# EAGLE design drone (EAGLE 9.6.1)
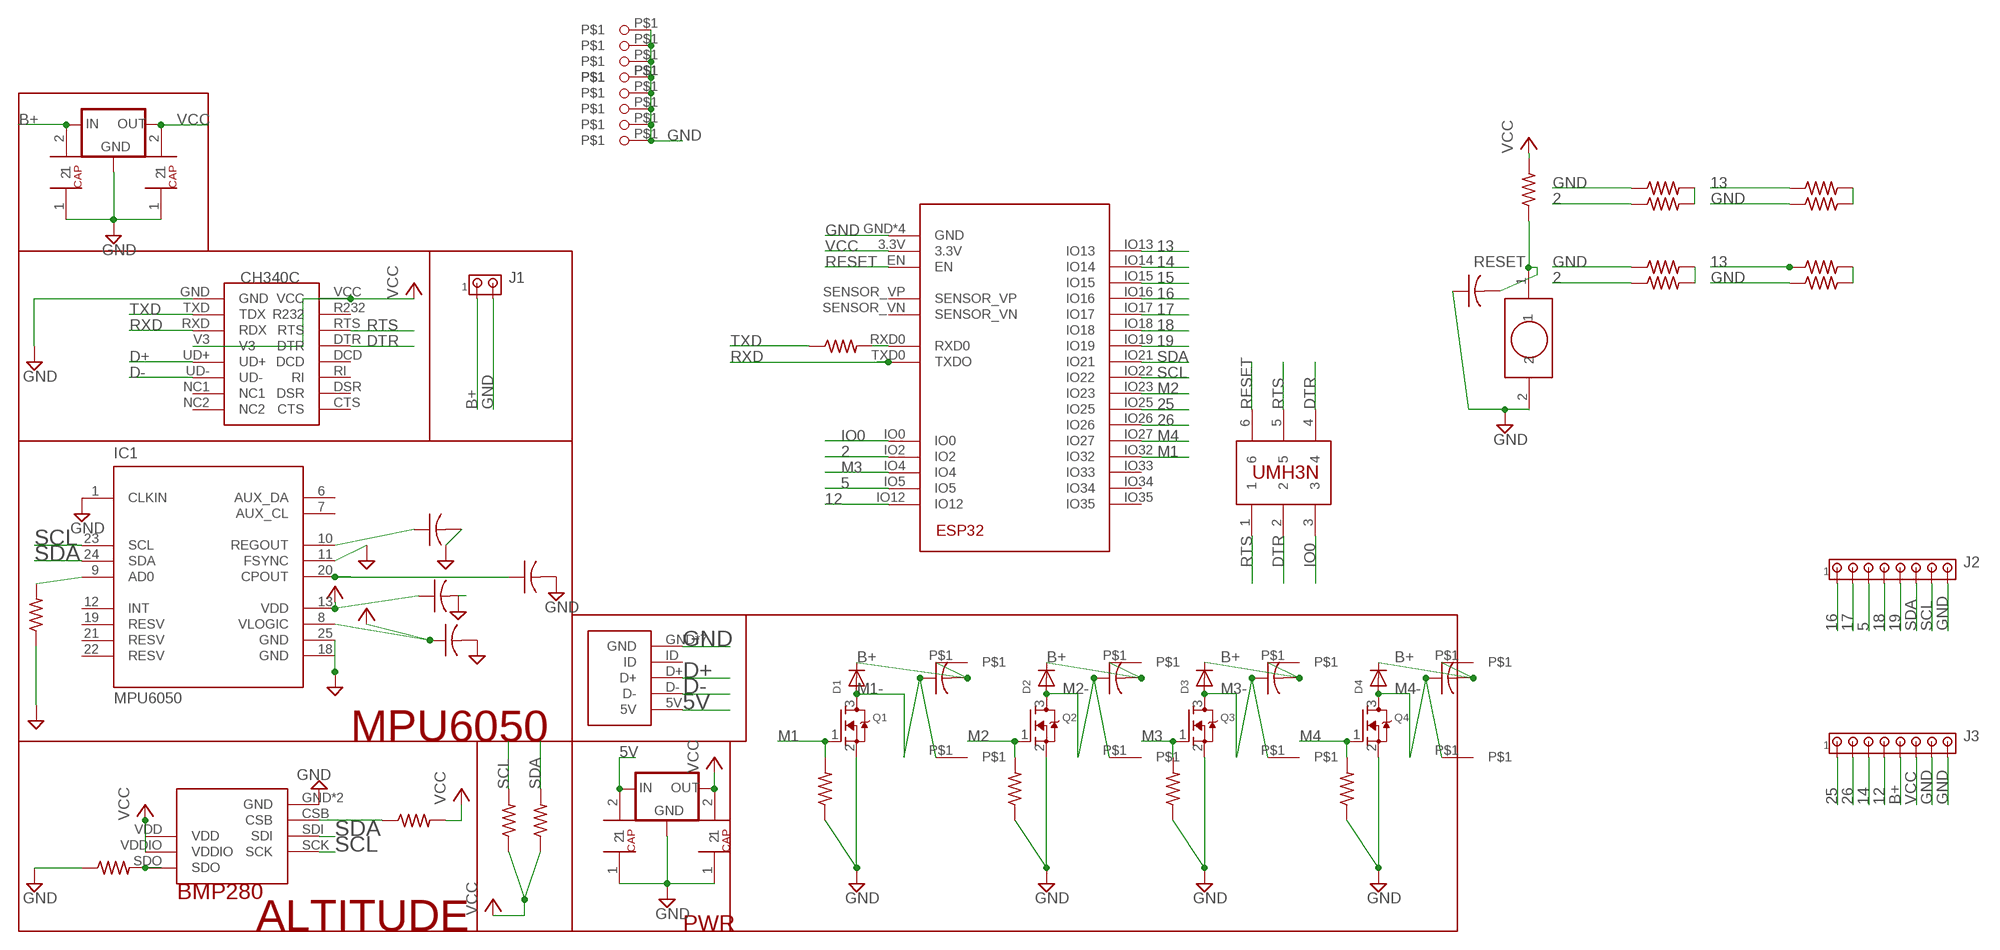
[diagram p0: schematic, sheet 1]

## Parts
D1  DIODESOD-323F  [SOD-323F]
D2  DIODESOD-323F  [SOD-323F]
D3  DIODESOD-323F  [SOD-323F]
D4  DIODESOD-323F  [SOD-323F]
IC1  MPU6050  [QFN50P400X400X95-25T265X275N]
IC2  SELF_VREG3.3MP  [SOT223]
IC3  SELF_VREG3.3MP  [SOT223]
J1  MTA02-100  [10X02MTA]
J2  MTA08-100  [10X08MTA]
J3  MTA08-100  [10X08MTA]
Q1  MOSFET-NREFLOW  [SOT23]
Q2  MOSFET-NREFLOW  [SOT23]
Q3  MOSFET-NREFLOW  [SOT23]
Q4  MOSFET-NREFLOW  [SOT23]
U1  ESP32  [MODULE_ESP-WROOM-32]
U$1  MICROUSB  [USB]
U$2  CH340C  [SOIC16]
U$3  BMP280  [BMP280]
U$4  R-US_R0603  [R0603]
U$5  R-US_R0603  [R0603]
U$6  C-USC0603  [C0603]
U$7  R-US_R0603  [R0603]
U$8  C-USC0603  [C0603]
U$9  C-USC0603  [C0603]
U$10  C-USC0603  [C0603]
U$11  R-US_R0603  [R0603]
U$12  R-US_R0603  [R0603]
U$13  SELF_CAP_0603SELF_CAP_0805  [SELF_CAP_0805]
U$14  SELF_CAP_0603SELF_CAP_0805  [SELF_CAP_0805]
U$16  R-US_R0603  [R0603]
U$18  SELF_CAP_0603SELF_CAP_0805  [SELF_CAP_0805]
U$19  SELF_CAP_0603SELF_CAP_0805  [SELF_CAP_0805]
U$20  R-US_R0603  [R0603]
U$21  R-US_R0603  [R0603]
U$22  R-US_R0603  [R0603]
U$23  R-US_R0603  [R0603]
U$24  C-USC0603  [C0603]
U$25  C-USC0603  [C0603]
U$26  C-USC0603  [C0603]
U$27  C-USC0603  [C0603]
U$28  UMH3N  [UMH3N]
U$29  SELF_PUSHBUTTON  [SELF_PUSHBUTTON]
U$30  R-US_R0603  [R0603]
U$31  C-USC0603  [C0603]
U$32  R-US_R0603  [R0603]
U$33  R-US_R0603  [R0603]
U$34  R-US_R0603  [R0603]
U$35  R-US_R0603  [R0603]
U$36  R-US_R0603  [R0603]
U$37  R-US_R0603  [R0603]
U$38  R-US_R0603  [R0603]
U$39  R-US_R0603  [R0603]
U$40  SELF_PINOUTS  [PINOUTS]
U$41  SELF_PINOUTS  [PINOUTS]
U$42  SELF_PINOUTS  [PINOUTS]
U$43  SELF_PINOUTS  [PINOUTS]
U$44  SELF_PINOUTS  [PINOUTS]
U$45  SELF_PINOUTS  [PINOUTS]
U$46  SELF_PINOUTS  [PINOUTS]
U$47  SELF_PINOUTS  [PINOUTS]
U$48  SELF_PIN2  [PIN2]
U$49  SELF_PIN2  [PIN2]
U$50  SELF_PIN2  [PIN2]
U$51  SELF_PIN2  [PIN2]
U$52  SELF_PIN2  [PIN2]
U$53  SELF_PIN2  [PIN2]
U$54  SELF_PIN2  [PIN2]
U$55  SELF_PIN2  [PIN2]
U$56  SELF_PIN2  [PIN2]

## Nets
2: U1.IO2 U$33.1 U$39.1
5: J2.3 U1.IO5
5V: IC2.VIN(IN) U$1.5V U$13.2
12: J3.4 U1.IO12
13: U1.IO13 U$34.1 U$36.1
14: J3.3 U1.IO14
15: U1.IO15
16: J2.1 U1.IO16
17: J2.2 U1.IO17
18: J2.4 U1.IO18
19: J2.5 U1.IO19
25: J3.1 U1.IO25
26: J3.2 U1.IO26
B+: D1.C D2.C D3.C D4.C IC3.VIN(IN) J1.1 J3.5 U$19.2 U$24.2 U$25.2 U$26.2 U$27.2 U$40.P$1 U$42.P$1 U$44.P$1 U$46.P$1
D+: U$1.D+ U$2.UD+
D-: U$1.D- U$2.UD-
DTR: U$2.DTR U$28.2 U$28.4
GND: IC1.1(CLKIN) IC1.11(FSYNC) IC1.18(GND) IC1.25(GND) IC2.GND IC3.GND J1.2 J2.8 J3.7 J3.8 Q1.2(S) Q2.2(S) Q3.2(S) Q4.2(S) U1.GND U1.GND1(GND) U1.GND2(GND) U1.GND3(GND) U$1.GND U$1.GND1(GND) U$1.GND2(GND) U$1.GND3(GND) U$1.GND4(GND) U$1.GND5(GND) U$1.GND6(GND) U$2.GND U$3.GND U$3.GND1(GND) U$5.1 U$6.2 U$7.1 U$8.2 U$9.2 U$10.2 U$13.1 U$14.1 U$18.1 U$19.1 U$20.1 U$21.1 U$22.1 U$23.1 U$29.2 U$31.1 U$32.1 U$35.1 U$37.1 U$38.1 U$48.P$1 U$49.P$1 U$50.P$1 U$51.P$1 U$52.P$1 U$53.P$1 U$54.P$1 U$55.P$1 U$56.P$1
IO0: U1.IO0 U$28.3
M1: Q1.1(G) U1.IO32 U$20.2
M1-: D1.A Q1.3(D) U$24.1 U$41.P$1
M2: Q2.1(G) U1.IO23 U$21.2
M2-: D2.A Q2.3(D) U$26.1 U$43.P$1
M3: Q3.1(G) U1.IO4 U$22.2
M3-: D3.A Q3.3(D) U$27.1 U$45.P$1
M4: Q4.1(G) U1.IO27 U$23.2
M4-: D4.A Q4.3(D) U$25.1 U$47.P$1
N$1: U$32.2 U$33.2
N$2: U$38.2 U$39.2
N$4: U$34.2 U$35.2
N$5: U$36.2 U$37.2
N$13: U$3.SDO U$5.2
N$14: U$3.CSB U$4.1
N$15: IC1.9(AD0) U$7.2
N$16: IC1.10(REGOUT) U$8.1
N$17: IC1.20(CPOUT) U$10.1
N$18: U1.RXD0 U$16.2
RESET: U1.EN U$28.6 U$29.1 U$30.1 U$31.2
RTS: U$2.RTS U$28.1 U$28.5
RXD: U1.TXD0(TXDO) U$2.RXD(RDX)
SCL: IC1.23(SCL) J2.7 U1.IO22 U$3.SCK U$11.2
SDA: IC1.24(SDA) J2.6 U1.IO21 U$3.SDI U$12.2
TXD: U$2.TXD(TDX) U$16.1
VCC: IC1.8(VLOGIC) IC1.13(VDD) IC2.VOUT1(OUT) IC2.VOUT(OUT) IC3.VOUT1(OUT) IC3.VOUT(OUT) J3.6 U1.3.3V U$2.V3 U$2.VCC U$3.VDD U$3.VDDIO U$4.2 U$6.1 U$9.1 U$11.1 U$12.1 U$14.2 U$18.2 U$30.2
Unconnected: IC1.2(NC) IC1.3(NC) IC1.4(NC) IC1.5(NC) IC1.6(AUX_DA) IC1.7(AUX_CL) IC1.12(INT) IC1.14(NC) IC1.15(NC) IC1.16(NC) IC1.17(NC) IC1.19(RESV) IC1.21(RESV) IC1.22(RESV) U1.IO33 U1.IO34 U1.IO35 U1.SENSOR_VN U1.SENSOR_VP U$1.ID U$2.CTS U$2.DCD U$2.DSR U$2.NC1 U$2.NC2 U$2.R232 U$2.RI

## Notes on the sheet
- MPU6050
- ALTITUDE | PWR

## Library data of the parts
D1-D4 = adafruit:DIODE: Diode
IC1 = invensense:MPU6050: The triple-axis MEMS gyroscope
IC2 IC3 = V_REG:SELF_VREG: 800mA Low-Dropout Linear Regulator Source: http://www.ti.com/lit/ds/symlink/lm1117-n.pdf; MF: Texas Instruments; MPN: LM1117MP-3.3; OC_FARNELL: 9778195; OC_NEWARK: 28X3416
J1 = con-amp:MTA02-100: AMP connector
J2 J3 = con-amp:MTA08-100: AMP connector
Q1-Q4 = adafruit:MOSFET-N: N-Channel Mosfet 2N7002E - 60V 260mA SOT23 [Digikey: 2N7002ET1GOSTR-ND] - REEL BSH103 - 30V 850mA SOT23 [Digikey: 568-5013-1-ND]
U1 = ESP-WROOM-32:ESP32: Module: combo; GPIO, I2C x2, I2S x2, SDIO, SPI x3, UART x3; 19.5dBm
U$1 = micro usb:MICROUSB
U$2 = ch340g:CH340C
U$3 = BMP280:BMP280
U$4 U$5 U$7 U$11 U$12 U$16 U$20-U$23 U$30 U$32-U$39 = rcl:R-US_: RESISTOR, American symbol; SPICEPREFIX: R
U$6 U$8-U$10 U$24-U$27 U$31 = rcl:C-US: CAPACITOR, American symbol; SPICEPREFIX: C
U$13 U$14 U$18 U$19 = SELF_CAP:SELF_CAP_0603
U$28 = UMH3N:UMH3N
U$29 = self_pushbutton:SELF_PUSHBUTTON
U$40-U$47 = PIN:SELF_PINOUTS
U$48-U$56 = PIN2:SELF_PIN2

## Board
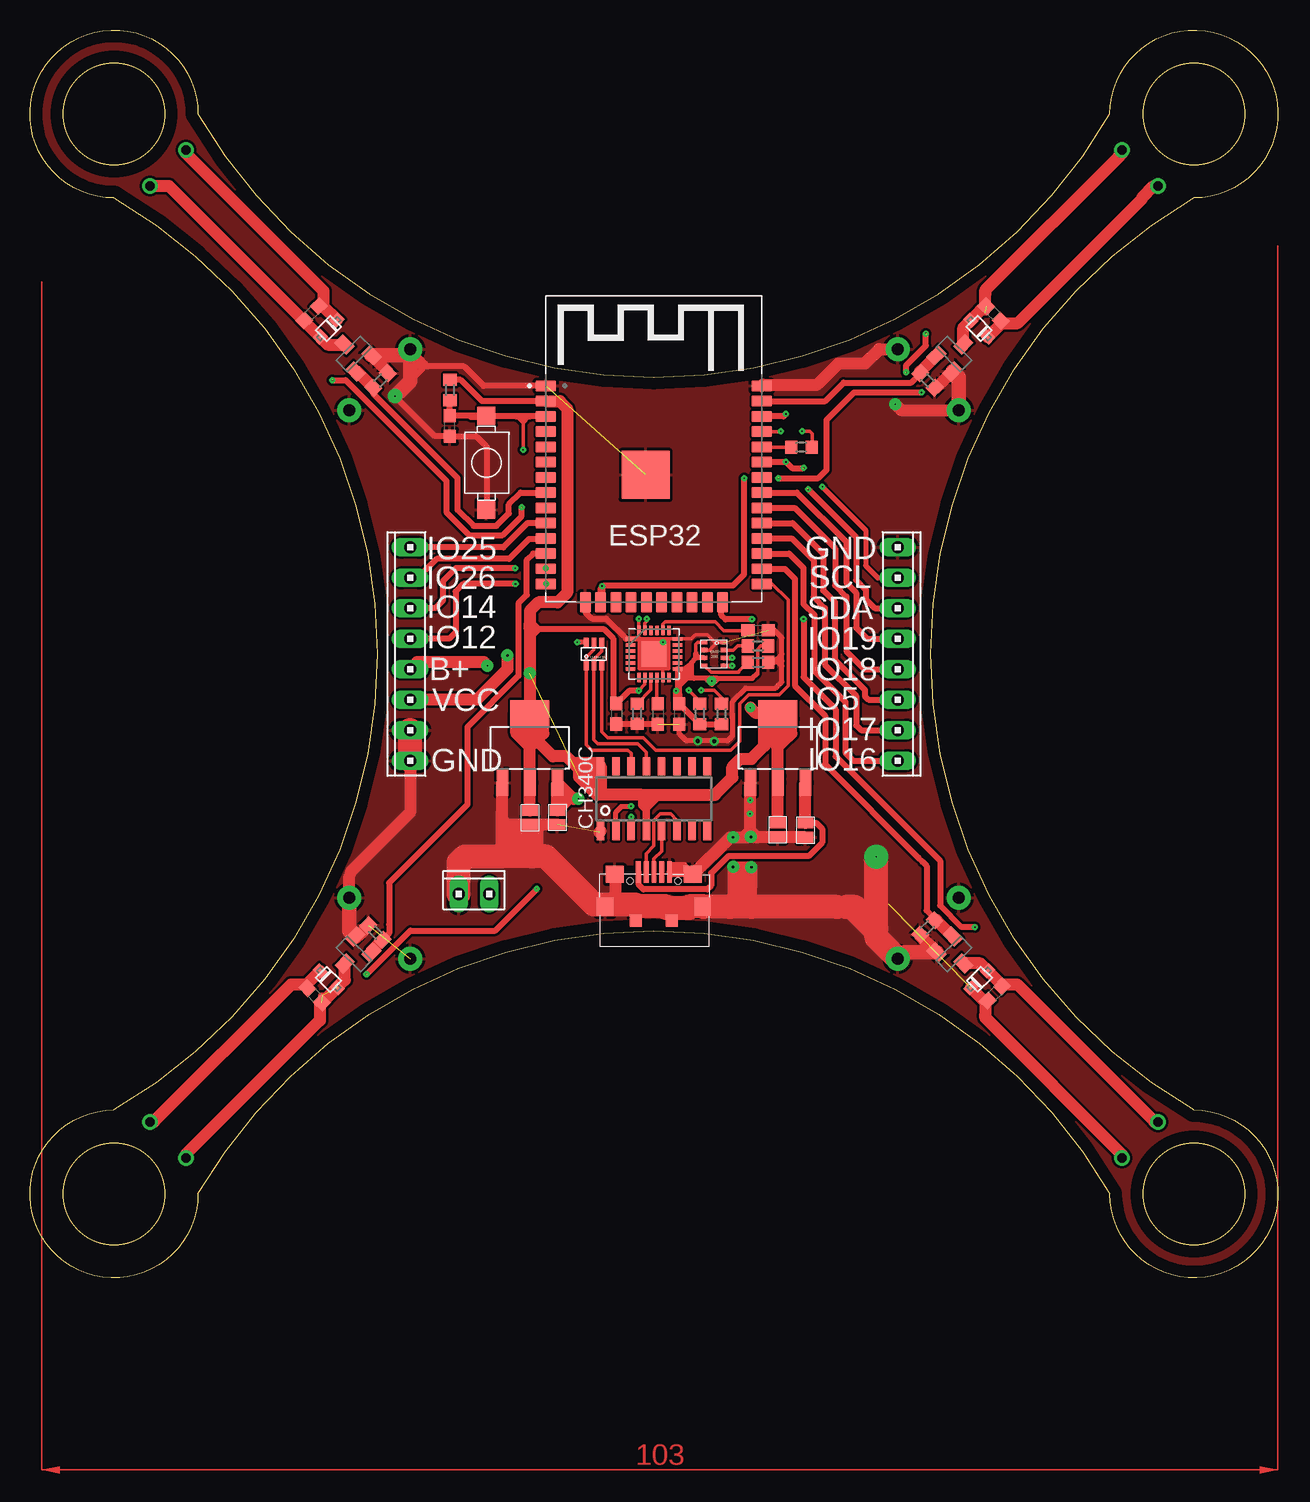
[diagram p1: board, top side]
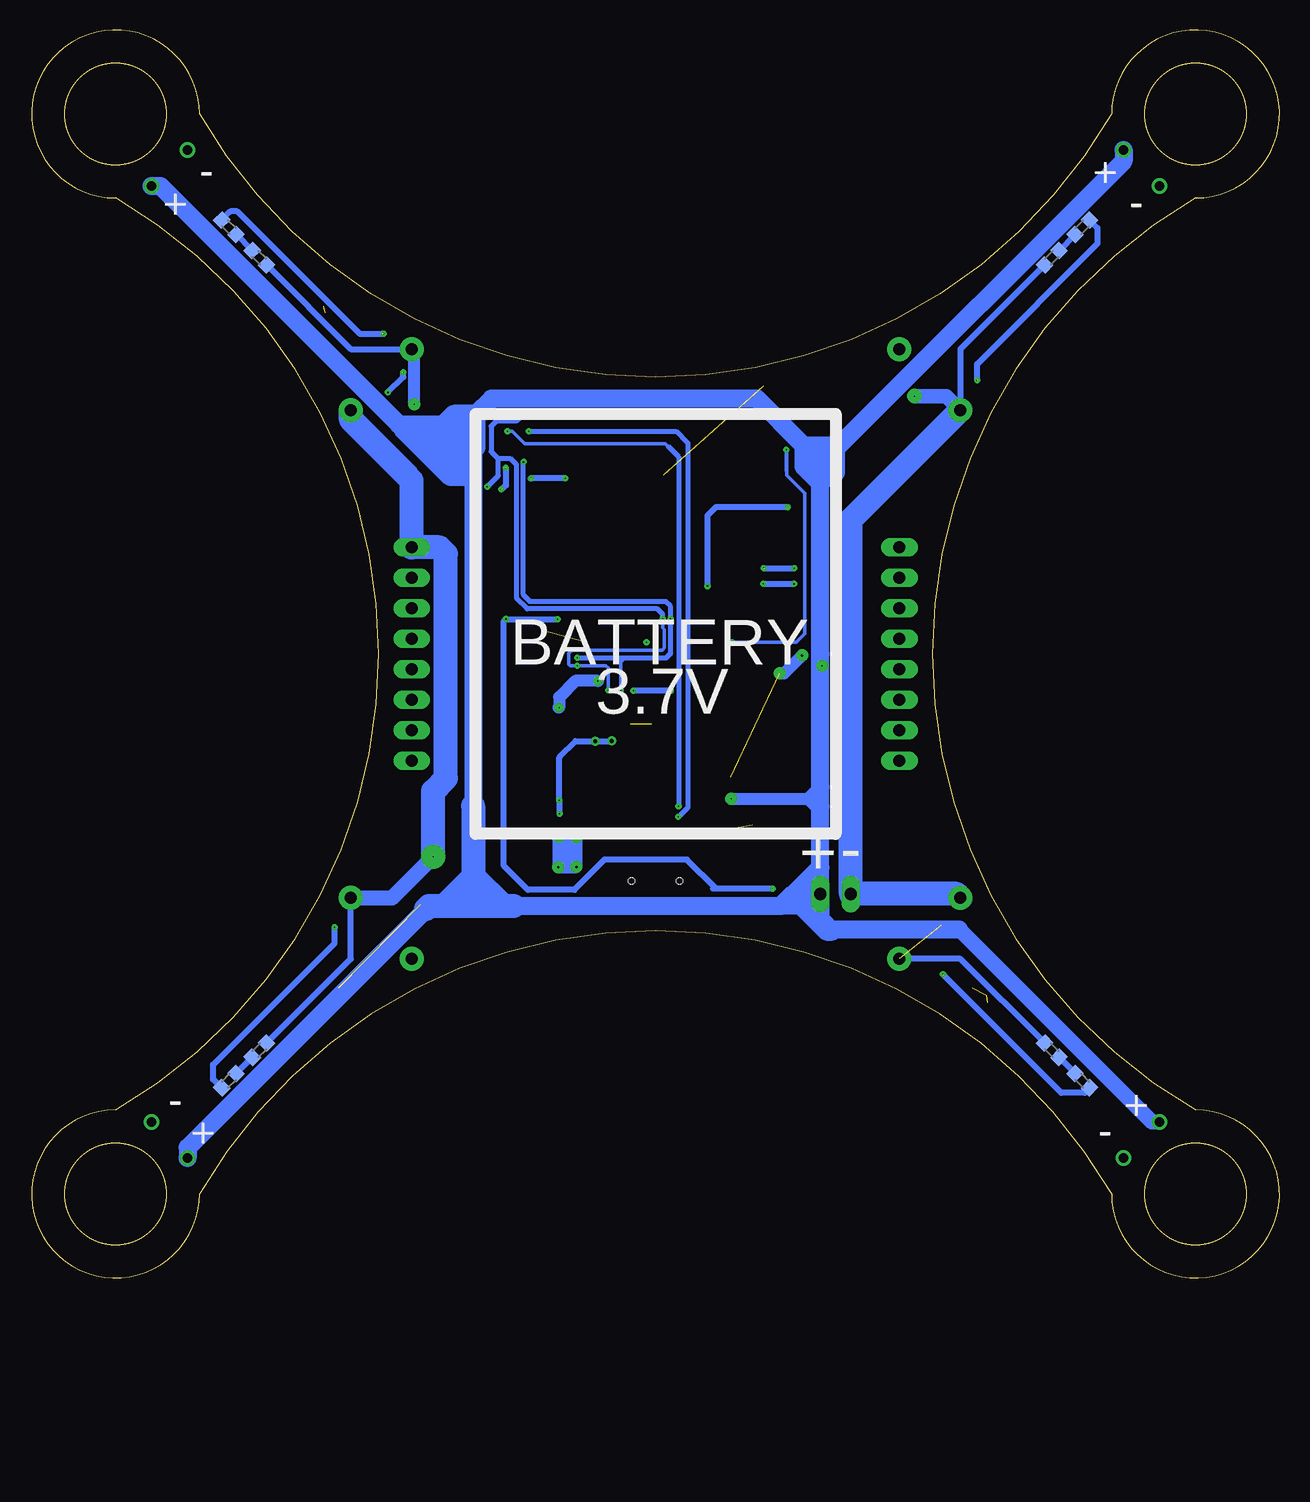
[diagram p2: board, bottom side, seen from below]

Size 103.99 x 103.99 mm. Coordinates in mm from the lower left corner, seen from the top.
Outline: 14,97 arc120 90,97 arc-270 97,90 arc120 97,14 arc-270 90,7 arc120 14,7 arc-270 7,14 arc120 7,90 arc-270 14,97
Outline: circle at 7,97 radius 4.25
Outline: circle at 7,7 radius 4.25
Outline: circle at 97,7 radius 4.25
Outline: circle at 97,97 radius 4.25
Copper layers (1*16): Top 0.035mm / dielectric 1.5mm / Bottom 0.035mm
Design rules "default *": minimum track width 6mil, minimum drill 0.35mm, track to track 6mil, track to pad 6mil, pad to pad 6mil, via to via 6mil, smd to smd 6mil, copper to edge 40mil, drill to drill 6mil, minimum pad ring 10mil, minimum via ring 8mil, stop-mask expansion 4mil, vias tented up to drill 10mm, thermal gap 10mil

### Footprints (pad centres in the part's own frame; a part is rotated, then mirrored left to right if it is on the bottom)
SOD-323F = smd 1 x 0.8: A -1,0; C 1,0
QFN50P400X400X95-25T265X275N = smd 0.26 x 0.79: 1 -1.25,-1.97; 2 -0.75,-1.97; 3 -0.25,-1.97; 4 0.25,-1.97; 5 0.75,-1.97; 6 1.25,-1.97; 13 1.25,1.97; 14 0.75,1.97; 15 0.25,1.97; 16 -0.25,1.97; 17 -0.75,1.97; 18 -1.25,1.97 | smd 0.79 x 0.26: 7 1.97,-1.25; 8 1.97,-0.75; 9 1.97,-0.25; 10 1.97,0.25; 11 1.97,0.75; 12 1.97,1.25; 19 -1.97,1.25; 20 -1.97,0.75; 21 -1.97,0.25; 22 -1.97,-0.25; 23 -1.97,-0.75; 24 -1.97,-1.25 | smd 2.15 x 2.05: 25 0,0
SOT223 = smd 0.95 x 2.15: GND -2.3,-2.9; VIN 2.3,-2.9; VOUT 0,-2.9 | smd 3.25 x 2.15: VOUT1 0,2.9
10X02MTA = drill 1.016 long: 1 1.27,0; 2 -1.27,0
10X08MTA = drill 1.016 long: 1 8.89,0; 2 6.35,0; 3 3.81,0; 4 1.27,0; 5 -1.27,0; 6 -3.81,0; 7 -6.35,0; 8 -8.89,0
SOT23 = smd 1 x 1.4: 1 -0.95,-1.1; 2 0.95,-1.1; 3 0,1.1
MODULE_ESP-WROOM-32 = smd 1.7 x 0.9: 3.3V -9,6.985; EN -9,5.715; GND -9,8.255; GND3 9,8.255; IO0 9,-8.255; IO4 9,-6.985; IO5 9,-3.175; IO12 -9,-8.255; IO14 -9,-6.985; IO16 9,-5.715; IO17 9,-4.445; IO18 9,-1.905; IO19 9,-0.635; IO21 9,1.905; IO22 9,5.715; IO23 9,6.985; IO25 -9,-3.175; IO26 -9,-4.445; IO27 -9,-5.715; IO32 -9,-0.635; IO33 -9,-1.905; IO34 -9,1.905; IO35 -9,0.635; NC 9,0.635; RXD0 9,3.175; SENSOR_VN -9,3.175; SENSOR_VP -9,4.445; TXD0 9,4.445 | smd 0.9 x 1.7: CLK 0.635,-9.755; CMD -0.635,-9.755; GND2 -5.715,-9.755; IO2 5.715,-9.755; IO13 -4.445,-9.755; IO15 4.445,-9.755; SD0 1.905,-9.755; SD1 3.175,-9.755; SD2 -3.175,-9.755; SD3 -1.905,-9.755 | smd 4 x 4: GND1 -0.7,0.845
USB = smd 0.4 x 1.8: 5V -1.298,0.204; D+ 0.002,0.204; D- -0.648,0.204; GND 1.302,0.204; ID 0.652,0.204 | smd 1.5 x 1.4: GND1 3.25,0; GND6 -3.25,0 | smd 1.35 x 1.5: GND2 4.075,-2.7; GND5 -4.075,-2.7 | smd 1 x 1: GND3 1.5,-3.85; GND4 -1.5,-3.85 | hole 0.5: -2,-0.55; 2,-0.55
SOIC16 = smd 0.635 x 1.524: CTS 4.445,2.695; DCD 0.635,2.695; DSR 3.175,2.695; DTR -0.635,2.695; GND -4.445,-2.695; NC1 3.175,-2.695; NC2 4.445,-2.695; R232 -3.175,2.695; RI 1.905,2.695; RTS -1.905,2.695; RXD -1.905,-2.695; TXD -3.175,-2.695; UD+ 0.635,-2.695; UD- 1.905,-2.695; V3 -0.635,-2.695; VCC -4.445,2.695
BMP280 = smd 0.5 x 0.35: CSB 0.8,0.325; GND 0.8,0.975; GND1 -0.8,0.325; SCK 0.8,-0.975; SDI 0.8,-0.325; SDO -0.8,-0.975; VDD -0.8,0.973; VDDIO -0.8,-0.325
R0603 = smd 1 x 1.1: 1 -0.85,0; 2 0.85,0
C0603 = smd 1.1 x 1: 1 -0.85,0; 2 0.85,0
SELF_CAP_0805 = smd 0.9 x 1.3: 1 0.6,0; 2 -0.6,0
UMH3N = smd 0.4 x 0.8: 1 -0.65,-0.97; 2 0,-0.97; 3 0.65,-0.97; 4 0.65,0.97; 5 0,0.97; 6 -0.65,0.97
SELF_PUSHBUTTON = smd 1.5 x 1.5: 1 0,3.9; 2 0,-3.9
PINOUTS = drill 0.8 pad 1.3: P$1 0,0
PIN2 = drill 1 pad 2: P$1 0,0

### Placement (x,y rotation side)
D1  24.89,79.11 45 top
D2  79.1,79.11 315 top
D3  79.11,24.89 225 top
D4  24.89,24.88 135 top
IC1  52,52 270 top
IC2  62.33,44.17 0 top
IC3  41.66,44.17 0 top
J1  37,32 0 top
J2  72.32,52 270 top
J3  31.68,52 90 top
Q1  26.99,77 45 top
Q2  76.99,77 315 top
Q3  77,27 224.4 top
Q4  27,26.99 135.4 top
U1  52,66.08 0 top
U$1  52,33.63 0 top
U$2  52,39.94 0 top
U$3  57,52 0 top
U$4  60.68,52.66 0 top
U$5  60.68,51.3 180 top
U$6  48.87,47.01 270 top
U$7  50.6,47.01 90 top
U$8  52.32,47 270 top
U$9  54.09,47 270 top
U$10  60.68,53.96 0 top
U$11  57.63,47 90 top
U$12  55.81,47 90 top
U$13  64.61,37.31 270 top
U$14  62.31,37.33 270 top
U$16  64.28,69.23 180 top
U$18  41.66,38.35 270 top
U$19  43.95,38.37 270 top
U$20  29.21,74.78 225 top
U$21  74.78,74.78 135 top
U$22  74.78,29.21 45 top
U$23  28.78,28.77 315 top
U$24  23.45,80.39 45 top
U$25  23.72,23.55 135 top
U$26  80.3,80.38 315 top
U$27  80.4,23.71 225 top
U$28  47,52 0 top
U$29  38.03,67.93 0 top
U$30  35,74 90 top
U$31  35,71 90 top
U$32  18.98,18.98 315 bottom
U$33  16.44,16.44 135 bottom
U$34  16.44,87.56 225 bottom
U$35  18.98,85.02 45 bottom
U$36  87.56,87.56 315 bottom
U$37  85.02,85.02 135 bottom
U$38  85.02,18.98 225 bottom
U$39  87.56,16.44 45 bottom
U$40  10,13 0 top
U$41  10,91 0 top
U$42  91,10 0 top
U$43  91,94 0 top
U$44  13,94 0 top
U$45  94,13 0 top
U$46  94,91 0 top
U$47  13,10 0 top
U$48  31.68,26.6 0 top
U$49  26.6,31.68 0 top
U$50  72.32,26.6 0 top
U$51  77.4,31.68 0 top
U$52  77.4,72.32 0 top
U$53  72.32,77.4 0 top
U$54  31.68,77.4 0 top
U$55  26.6,72.32 0 top
U$56  31.68,26.6 0 top

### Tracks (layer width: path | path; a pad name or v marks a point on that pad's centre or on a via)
2  (via drill 0.1 pad 0.5)  (2 unrouted)
  Top 0.508: v60.17,54.89 57.96,54.89 57.62,55.23 57.62,56.23 U1.IO2 | v64.46,54.91 64.46,50.06 67.14,47.38 67.14,43.46 75.84,34.77 75.84,31.01 77.62,29.23 v78.75,29.23 | v28.04,25.3 31.69,28.95 38.78,28.95 42.22,32.39
  Bottom 0.508: 78.75,29.14 78.75,27.9 88.86,17.78 88.86,16.54 U$39.1 | 78.75,29.14 78.75,29.15 | 78.75,29.14 v78.75,29.23 | v60.17,54.89 64.44,54.89 v64.46,54.91 64.63,54.73 64.63,34.33 62.64,32.34 58.77,32.34 56.26,34.85 50,34.85 49.62,34.85 49.39,34.85 47,32.45 | 28.03,25.28 18.17,15.41 16.26,15.41 U$33.1 | 47.22,32.45 47,32.45 | 47,32.45 42.26,32.45 v42.23,32.42
5
  Top 0.508: U1.IO5 63.54,62.9 66.1,60.34 66.1,57.3 67.06,56.34 67.06,51.52 69.57,49.01 69.57,48.48 69.86,48.19 J2.3
5V
  Top 0.5: U$13.2 65.54,37.91 66.02,37.43 66.02,36.28 64.89,35.15 58.19,35.15 56.76,33.72 56.76,32.69 56.46,32.38 51.13,32.38 50.7,32.81 U$1.5V
  Top 1: U$13.2 64.61,41.25 IC2.VIN
12  (via drill 0.1 pad 0.5)
  Top 0.508: U1.IO12 43,57.86 v43.01,57.86 | v40.46,57.83 36.12,57.83 35.47,57.18 35.47,53.81 34.92,53.27 J3.4
  Bottom 0.508: v43.01,57.86 40.48,57.86 v40.46,57.83
13  (via drill 0.1 pad 0.5)  (5 unrouted)
  Top 0.508: v59.52,66.63 59.52,58.63 58.59,57.7 47.83,57.7 47.55,57.43 U1.IO13 47.67,56.44 v47.67,57.65 | v62.37,66.65 65.71,66.65 66.39,67.33 66.39,71.51 68.68,73.8 74.28,73.8 v74.3,73.79 | v73.02,75.46 73.02,76.04 74.66,77.69 v74.66,78.69 | v25.2,74.82 26.3,74.82 34.7,66.42 34.7,63.82 36.62,61.89 39.38,61.89 40.98,63.49 40.98,64.17
  Bottom 0.508: 74.76,78.69 76.67,78.69 86.86,88.88 87.43,88.88 U$36.1 | v59.52,66.63 62.41,66.63 | v74.3,73.79 73.02,75.07 73.02,75.44 | v40.98,64.23 46.96,64.23 47.67,63.52 v47.67,57.65 | U$34.1 15.15,87.48 15.15,86.2 25.2,76.16 25.2,74.86
14  (via drill 0.1 pad 0.5)  (1 unrouted)
  Top 0.508: v40.44,59.15 35.5,59.15 34.41,58.05 34.41,56.43 33.78,55.81 J3.3
  Bottom 0.508: v42.99,59.15 v40.44,59.15
16
  Top 0.508: U1.IO16 63.26,60.36 64.45,59.17 64.45,56.16 65.36,55.25 65.36,50.58 67.94,48 67.94,43.78 68.62,43.11 J2.1
17
  Top 0.508: U1.IO17 63.48,61.63 65.3,59.81 65.3,56.74 66.24,55.81 66.24,51.12 68.85,48.5 68.85,46.05 69.25,45.65 J2.2
18
  Top 0.508: U1.IO18 63.71,64.17 67.09,60.8 67.09,57.7 68.02,56.77 68.02,52.24 69.53,50.73 J2.4
19
  Top 0.508: U1.IO19 63.91,65.44 68.02,61.33 68.02,57.94 68.85,57.12 68.85,54.18 69.77,53.27 J2.5
25
  Top 0.508: U1.IO25 41.46,62.9 39.44,60.89 J3.1
26
  Top 0.508: U1.IO26 42.93,61.57 41.58,61.57 39.93,59.92 33.9,59.92 32.37,58.39 32.37,58.32 31.7,58.32 J3.2
B+  (via drill 0.1 pad 1)  (1 unrouted)
  Top 0.203: U$27.2 79.77,23.14 79.61,22.97 | U$25.2 23.24,24.21 23.02,24.43 | U$26.2 80.82,79.73 80.98,79.57
  Top 1: IC3.VIN 43.95,41.25 43.95,39.92 U$19.2 | D4.C 23.02,24.43 21.84,24.43 | D2.C 80.98,79.57 82.29,79.57 | D3.C 79.61,22.97 79.61,22 79.61,21.67
  Top 1.016: v45.7,39.92 43.95,39.92 | v45.7,39.92 45.28,39.92 43.95,41.25 | v45.7,39.92 44.9,39.92 U$19.2 | v38.12,51.02 37.83,51.31 32.26,51.31 J3.5 | 21.84,24.43 21.76,24.43 10.32,13 U$40.P$1 | 79.61,22 79.61,21.67 91,10.28 U$42.P$1 | U$44.P$1 13,93.72 24.45,82.26 24.45,81.03 24.42,80.99 | 82.29,79.57 92.67,89.94 92.67,90 93.66,91 U$46.P$1 | D1.C 24.42,80.99 | 24.42,80.99 U$24.2
  Bottom 0.5: 71.13,31.56 71.55,31.13
  Bottom 1.016: v45.7,39.92 39.3,39.92 | 39.3,39.92 38.89,39.92 38.27,39.3 38.67,39.3 39.3,39.92 | 39.3,39.92 38.29,40.92 38.27,40.92 | v38.12,51.02 38.12,51.85 38.27,52
  Bottom 1.27: 26.7,29.04 26.68,29.04 10.63,13 U$40.P$1
  Bottom 1.5: J1.1 38.27,29.38 | 38.27,29.38 37.77,28.88 | 37.77,28.88 37.76,28.87 37.26,28.87 37.44,29.04 | 37.44,29.04 26.7,29.04 | J1.1 40.34,32 | 63.85,31 41.55,31 | J1.1 38.27,34.22 | 38.27,34.22 38.27,39.3 38.27,40.92 38.27,52 38.27,66.23 | 38.27,66.23 38.27,67.24 | 38.27,67.24 38.27,68.08 | 38.27,68.08 36.96,69.39 | 67.19,66.73 67.19,39.31 | 71.69,69.32 73.14,70.77 73.04,70.77 | 38.27,68.08 38.36,68.08 39.67,69.4 | 39.67,69.4 43.54,73.27 65.66,73.27 66.93,72.01 | 68.2,70.74 66.93,72.01 | 68.2,70.74 69.62,69.32 | 69.62,69.32 71.69,69.32 | 68.2,70.74 68.2,69.28 | 68.2,69.28 68.2,67.95 67.19,68.96 | 67.19,68.96 67.19,66.73 | 39.67,69.4 36.98,69.4 36.96,69.39 | 36.96,69.39 36.96,69.1 | 36.96,69.1 36.96,67.11 37.4,66.67 37.7,66.67 38.27,67.24 | 39.67,69.4 39.67,67.64 38.27,66.23 | 38.27,34.22 40.34,32.14 40.34,32 | 40.34,32 39.34,31 | 37.77,28.88 37.77,29.43 39.34,31 | 38.27,29.38 39.34,30.45 | 39.34,30.45 39.34,31 | 39.34,31 39.89,31 | 39.34,30.45 39.89,31 | 39.89,31 41.55,31 | 40.34,32 40.55,32 41.55,31 | 37.44,29.04 38.27,29.87 J1.1 | 71.13,30.74 91,10.87 U$42.P$1 | 66.93,72.01 66.93,70.55 | 66.93,70.55 68.2,69.28 | 66.93,70.55 66.93,69.22 67.19,68.96 | 67.19,66.73 69.62,69.16 69.62,69.32 | 67.19,66.73 69.1,66.73 71.69,69.32 | 66.93,72.01 68.83,72.01 69.71,71.13 | 69.71,71.13 70.81,70.02 71.19,70.02 72.14,70.98 | 72.14,70.98 | 72.14,70.98 72.35,70.77 73.04,70.77 | 73.04,70.77 73.41,71.13 | 73.41,71.13 69.71,71.13 | U$44.P$1 13,93.07 36.96,69.1 | 73.41,71.13 93.27,91 U$46.P$1
  Bottom 2: 71.13,30.74 70.86,31 69.21,31 | 69.21,31 67.26,31 | 67.26,31 64.7,31 | 64.7,31 63.85,31 | 67.19,39.31 67.19,33.44 | 67.19,33.44 67.19,31.07 67.26,31 | 64.7,31 67.14,33.44 67.19,33.44 | 67.19,33.44 69.21,31.42 69.21,31
D+
  Top 0.305: U$1.D+ 52,34.92 52.63,35.55 U$2.UD+
D-
  Top 0.254: 51.36,33.85 U$1.D-
  Top 0.305: U$1.D- 51.35,35.36 52,36.01 52,38.12 52.54,38.66 53.38,38.66 53.9,38.15 U$2.UD- 53.9,37.65
DTR
  Top 0.305: U$28.4 47.65,52.22 47,51.57 U$28.2 47,44.83 47.32,44.5 50.66,44.5 51.36,43.81 U$2.DTR
GND  (via drill 0.1 pad 0.4, 0.1 pad 1, 0.1 pad 1.2, 0.1 pad 2, 0.2 pad 1, 0.35)  (5 unrouted)
  Top 0.3: 57.28,52.97 57.07,52.97 | IC1.18 55.09,53.25 55.44,53.59 56.45,53.59 57.07,52.97 | 56.69,52.38 56.96,52.65 57.07,52.76 57.07,52.97
  Top 0.305: U$3.GND1 56.63,52.32 56.69,52.38 | 56.96,52.65 57.28,52.97 U$3.GND | IC1.11 52.75,50.75 53,51 IC1.25 51,52 51,53 | IC1.18 IC1.1 | 48.77,32 48.77,30.93 | U$1.GND2 54.65,30.93 53.82,30.1 52.92,30.1 | U$1.GND3 52.53,30.75 52.53,30.93 | U$1.GND4 50.42,29.86 50.42,31.11 | 49.31,31.11 48.1,31.11 U$1.GND5 50.49,30.93 50.54,30.98 47.68,30.98 | 47.68,30.98 47.14,30.98 47.02,31.11 | 49.26,31.31 48,31.31 47.68,30.98
  Top 0.4: IC1.25 52,52.22 v52.75,52.97 | 58.54,46.6 58.54,47 58.54,48.05 59.63,49.14 62.15,49.14 62.5,49.5 | v60.01,39.8 60.01,41.25 IC2.GND 60,41.24 v60,38.67
  Top 0.406: 58.54,47 58.54,45.15 58.14,44.75 v55.65,44.75 54.7,44.75 54.09,45.36 U$9.2 | 62.5,49.5 62.65,49.65 62.65,51 | 62.65,51 62.65,51.4 | 62.65,51.4 62.65,51.99 | 62.65,51.99 62.65,53.34 62,54 61.56,54 U$10.2 | U$5.1 62,51.3 | 62,51.3 62.35,51.3 62.65,51 | 62,51.3 62.1,51.4 62.65,51.4 | 62,51.3 62,51.33 62.65,51.99
  Top 0.45: 51,53 50.75,53.25 IC1.1 49.68,53.25
  Top 0.5: U1.GND2 46.28,55.49 46.83,54.94 47.98,54.94 49.68,53.25
  Top 0.508: U$29.2 38.05,64.05 38.05,69.27 37.17,70.15 U$31.1 33.74,70.15 v30.41,73.48 | U1.GND 37.8,74.33 36.17,75.96 33.13,75.96 | 32.51,76.58 31.7,77.4 U$54.P$1 | 32.9,76.2 33.13,75.96 | 33.13,75.96 32.9,75.96 | 30.96,74.03 32.9,75.96 | 32.9,75.96 32.14,75.96 | 32.14,75.96 31.83,75.96 31.68,76.12 | 32.9,75.96 32.9,76.2 | 32.9,76.2 32.51,76.58 | 32.51,76.58 32.51,76.33 32.14,75.96 | U$1.GND1 53.5,33.63 U$1.GND 54.01,33.83 | U$1.GND1 55.04,33.83 54.38,33.83 | 54.38,33.83 54.01,33.83 | U$1.GND1 54.54,34.33 54.54,34.39 54,34.39 | 54,34.39 53.5,34.39 53.5,34.34 54.01,33.83 | 54,34.39 54.38,34.01 54.38,33.83 | U$6.2 U$7.1 52.3,46.16 U$8.2 | U$9.2
  Top 1: U$18.1 | U$13.1 62.34,36.71 U$14.1 60.57,36.73 | U$19.1 43.94,37.75 42.31,37.75 U$18.1 | U$18.1 41.2,37.75 40.46,37.75 39.76,37.75 39.33,38.18 39.33,38.77 39.33,41.24 IC3.GND | IC2.GND 60.03,37.27 60.57,36.73 | 60.58,36.72 60.57,36.73
  Top 1.016: v72.09,72.81 72.59,72.32 U$52.P$1 | U1.GND3 61.1,74.44 65.6,74.44 67.38,76.22 69.58,76.22 70.76,77.4 U$53.P$1 | J3.8 31.68,38.79 26.79,33.9 26.6,33.38 U$49.P$1 | 43.95,37.75 43.94,37.75 | 47.44,37.13 U$2.GND | 43,35.13 42.31,35.82 42.31,37.75 | 41.62,36.98 41.73,37.09 41.84,36.99 41.84,35.13 41.2,35.77 41.2,37.75 | 40.46,36.29 39.3,35.13 39.3,38.74 39.33,38.77 | 40.46,36.29 40.46,37.75 | 39.76,37.75 39.76,36.99 40.46,36.29 | 49.46,31.31 49.26,31.31 | 47.02,31.11 46.92,31.21 | U$1.GND5 47.33,31.52 | 60.58,36.72 59.72,36.72 | 60.09,34.24 v60.11,34.22 | 60.03,37.27 60.03,36.81 v60.08,36.75 59.72,36.75 | 59.72,36.75 59.72,36.94 | 59.72,36.72 59.72,36.75 | 58.32,30.93 58.59,31.2 v58.59,34.24 58.61,34.22 v60.11,34.22 | v60.11,34.22 60.11,30.96 60.14,30.93 | v60.11,34.22 60.11,32.68 59.2,31.77 | v60.11,34.22 59.11,33.22 59.11,32.51 | U$1.GND1 58.34,36.72 v58.59,36.72 59.72,36.72 | Q1.2 29.81,75.52 U$20.1 | Q2.2 75.52,74.18 U$21.1 | Q3.2 74.18,28.49 U$22.1 | U$23.1 27.25,28.44 Q4.2 | U$1.GND6 48.77,33.61 48.77,32
  Top 1.2: v30.41,73.48 30.96,74.03 31.68,74.74 31.68,76.12 U$54.P$1 31.17,76.89 Q1.2 | Q4.2 26.6,28.94 U$49.P$1 | Q3.2 72.84,27.12 U$50.P$1 | Q2.2 77.4,75.04 U$52.P$1
  Top 1.27: U$1.GND2 52.53,30.93 48.77,30.93 U$1.GND5 | 67.24,30.93 67.98,30.93 U$50.P$1
  Top 2: J1.2 35.73,34.62 36.24,35.13 39.3,35.13 41.84,35.13 43,35.13 47.02,31.11 49.31,31.11 50.42,31.11 50.54,30.98 52.89,30.98 53.06,30.81 54.94,30.81 55.1,30.98 56.03,30.98 56.07,30.94 56.14,30.93 58.32,30.93 60.14,30.93 67.24,30.93 | U$50.P$1 70.53,28.39 70.53,29.14 | 70.53,29.14 v70.53,35.11 | 70.53,29.14 68.73,30.93 67.98,30.93 | J3.8 J3.7
  Bottom 0.5: 60.02,39.81 v60.01,39.8 60,39.78 v60,38.67
  Bottom 0.508: U$51.P$1 77.4,26.6 U$38.1 | U$53.P$1 77.4,77.4 U$37.1 | U$55.P$1 26.6,77.4 U$35.1 | U$32.1 26.6,26.6 U$48.P$1 | v60.01,39.8 60.01,43.38 58.66,44.74 v57.03,44.74 v57.03,44.73 55.67,44.73 v55.65,44.75
  Bottom 1.016: U$52.P$1 72.32,67.24 J2.8 | J2.8 | v72.09,72.81 72.09,77.17 U$53.P$1 | v58.59,36.72 v58.59,34.25 | v58.59,34.25 v58.59,34.24 | v58.59,34.25 58.61,34.22 v60.11,34.22 60.11,36.72 v60.08,36.75 | v60.08,36.75 58.62,36.75 v58.59,36.72 | v60.08,36.75 60.08,35.73 | 60.08,35.73 59.32,34.96 59.32,35.99 v58.59,36.72 | v58.59,36.72 59.09,36.72 60.08,35.73
  Bottom 1.2: U$55.P$1 27.76,73.48 v30.41,73.48
  Bottom 1.27: U$51.P$1 73.96,31.68 v70.53,35.11
  Bottom 2: U$55.P$1 35.73,63.19 J1.2 26.92,32 U$49.P$1 | v70.53,35.11 70.53,40.57 69.46,41.64 69.46,60.33 70.02,60.89 J2.8 72.32,66.44 77.4,71.52 U$52.P$1
  pour Top (isolate 0.2): -1.34,-1.34 -1.34,105.34 105.34,105.34 105.34,-1.34
IO0
  Top 0.3: U1.IO0 61.7,57.82 61.78,57.91 63.17,56.52 63.17,49.33 62.42,48.58 59.88,48.58 59.14,47.84 59.14,45.82 | 47.63,51.01 47.63,45.52 48.07,45.08
  Top 0.305: 47.69,50.98 U$28.3 47.63,51.01 | 61.07,57.9 U1.IO0 | 48.07,45.08 48.13,45.02 51.1,45.02 52.16,43.96 58.39,43.96 59.14,44.71 59.14,45.82
M1
  Top 0.508: U1.IO32 40.89,65.44 39.91,64.46 39.91,63.71 38.87,62.67 36.96,62.67 35.64,63.99 35.64,66.65 29.02,73.27 29.01,73.27 28.61,73.67 U$20.2
  Top 1.016: Q1.1 27.24,75.55 U$20.2
M1-
  Top 1: D1.A 24.8,77.78 Q1.3
  Top 1.016: 10.28,91 U$41.P$1 11.58,91 22.85,79.73 | D1.A 22.85,79.73 | 22.85,79.73 U$24.1
M2
  Top 0.508: U1.IO23 66.26,73.06 67.8,74.6 73.44,74.6 74.18,75.34 U$21.2
  Top 1.016: Q2.1 74.18,75.53 U$21.2
M2-  (1 unrouted)
  Top 0.203: U$26.1 80.03,80.65 79.23,80.65
  Top 0.508: 79.72,80.44 79.56,80.44
  Top 1: Q2.3 77.77,79.19 D2.A 79.23,80.65 79.62,81.04 79.62,82
  Top 1.016: 79.62,82 79.62,82.33 90.73,93.44 90.75,93.44 91,93.68 U$43.P$1
M3
  Top 0.508: U1.IO4 62.91,59.09 63.74,58.26 63.74,49.36 66.25,46.85 66.25,42.81 74.03,35.03 74.39,34.67 74.72,34.34 74.72,30.64 75.54,29.82
  Top 1.016: Q3.1 75.54,29.82 U$22.2
M3-
  Top 0.203: U$27.1 80.86,24.45 80.96,24.45
  Top 0.508: 78,26.21 Q3.3
  Top 1: 82.08,24.45 80.96,24.45 D3.A 79.2,26.21 78,26.21
  Top 1.016: 82.08,24.45 82.26,24.45 93.71,13 U$45.P$1
M4
  Top 0.508: U1.IO27 41.92,60.36 41.41,59.85 41.41,56.93 40.7,56.22 40.7,50.17 36.44,45.91 36.44,39.44 29.92,32.92 29.92,29.46 29.92,28.71 U$23.2
  Top 1.016: U$23.2 28.45,27.24 Q4.1
M4-  (2 unrouted)
  Top 0.203: U$25.1 24.45,23.67 24.76,23.35
  Top 0.508: 24.27,23.55 24.4,23.55
  Top 1: Q4.3 26.24,26.19 26.24,24.84 24.76,23.35 24.17,22.76 24.17,22
  Top 1.016: U$47.P$1 13,10.29 24.17,21.46 24.17,22
N$1
  Bottom 0.508: U$33.2 U$32.2
N$2
  Bottom 0.508: U$39.2 U$38.2
N$4
  Bottom 0.508: U$35.2 U$34.2
N$5
  Bottom 0.508: U$37.2 U$36.2
N$13
  Top 0.305: U$3.SDO 56.75,50.47 59,50.47 | 59,50.47 59.06,50.47 | 59,50.47 U$5.2
N$14
  Top 0.305: U$4.1 58.96,52.66 58.62,52.32 U$3.CSB
N$15
  Top 0.305: IC1.9 51.75,49 U$7.2
N$16
  Top 0.305: IC1.10 52.25,47.92 U$8.1
N$17
  Top 0.305: IC1.20 52.75,54.49 52.93,54.67 56,54.67 56.27,54.67 57.09,54.67 57.83,53.94 59.8,53.94 U$10.1
N$18
  Top 0.305: U$16.2 61.02,69.23 U1.RXD0
  Top 0.508: 60.97,69.25 U1.RXD0
RESET  (via drill 0.1 pad 0.3)
  Top 0.3: v45.62,52.97 v45.61,52.97 | 41.09,71.23 41.09,71.74 41.04,71.79 | v41.09,69.01 41.09,71.23 | 41.09,71.23 41.66,71.79 | 41.09,71.23 40.52,71.79 40.49,71.79
  Top 0.4: U$28.6 v45.62,52.97
  Top 0.508: U$29.1 38.06,71.79 40.49,71.79 41.04,71.79 41.66,71.79 U1.EN | U$29.1 37.95,71.75 36.74,71.75 | U$30.1 U$31.2 35.02,71.83 U$29.1
  Bottom 0.3: v45.61,52.97 40.27,52.97 39.56,53.69 39.56,65.39 41.06,66.89 41.06,67.24 | 41.06,67.24 41.06,68.97 | v41.09,69.01 41.09,67.27 41.06,67.24
RTS
  Top 0.305: U$28.5 47,52.36 46.35,51.71 U$28.1 46.35,44.42 46.8,43.96 49.83,43.96 50.09,43.7 U$2.RTS
RXD  (via drill 0.1 pad 0.4)
  Top 0.305: v62.57,70.55 62.55,70.52 U1.TXD0
  Top 0.4: U$2.RXD 50.1,37.26 v50.1,38.43
  Top 0.508: U1.TXD0 60.98,70.52
  Bottom 0.4: v62.57,70.55 50.29,70.55 49.31,69.57 49.31,39.19 50.07,38.43 v50.1,38.43
SCL  (via drill 0.1 pad 0.3, 0.1 pad 0.5)
  Top 0.305: IC1.23 51.25,54.57 51.41,54.73 v51.41,54.94 | 61.25,71.79 U1.IO22 | v55.94,48.97 56.6,48.97 56.62,48.95 57.04,48.95 58,48 57.85,47.85 U$11.2
  Top 0.4: U$3.SCK v58.51,51.02 | v58.51,51.02
  Top 0.406: v66.04,65.92 69.64,62.32 69.64,59.35 70.65,58.34 J2.7
  Top 0.508: v63,72 62.79,71.79 61.25,71.79
  Bottom 0.305: 51.41,54.54 51.41,54.18 51.25,54.02 51.25,52.5 51.44,52.32 58.95,52.32 59.21,52.05 59.21,51.14 59.09,51.02 v58.51,51.02 58.51,51.03 56.13,51.03 55.94,50.84 v55.94,48.97 | v51.41,54.93 v51.41,54.94 | 65.71,68.86 65.66,68.82
  Bottom 0.406: v66.04,65.92 65.1,66.85 65.1,68.26 | 65.66,68.82 65.1,68.26 | 65.71,68.86 65.71,70.98 65.23,71.45 63.54,71.45 v63,72 | 65.1,68.26 64.08,68.26 63.61,67.79 63.61,56.65 62.71,55.75 51.85,55.75 51.41,55.31 v51.41,54.93 51.41,54.54
SDA  (via drill 0.1 pad 0.3, 0.1 pad 0.5)  (2 unrouted)
  Top 0.305: v50.74,54.94 v50.75,54.94 IC1.24 | 61.21,67.98 U1.IO21 | v54.9,48.96 55.81,48.04 U$12.2
  Top 0.4: U$3.SDI v58.52,51.67
  Top 0.508: 64.44,67.49 63.51,67.49 v63,68 62.98,67.98 61.21,67.98 | v64.86,65.7 68.85,61.71 68.85,58.18 69.67,57.36 69.67,56.54 70.4,55.81 J2.6
  Bottom 0.305: v58.52,51.67 55.17,51.67 | 55.17,51.67 55,51.67 | 55,51.67 54.54,51.67 | 54.54,51.67 52,51.67 | 62.44,56.36 62.66,56.57 | 63.02,67.97 v63,68 | v54.9,48.96 54.9,51.32 | 54.9,51.32 54.9,51.58 55,51.67 | 54.54,51.67 54.9,51.32 | 54.9,51.32 55.17,51.59 55.17,51.67
  Bottom 0.406: 62.66,56.57 63.02,56.93 63.02,56.94 | 63.02,67.97 63.02,56.94 62.44,56.36 51.15,56.36 50.74,55.96 v50.74,54.94 50.74,52.04 51.11,51.67 52,51.67 55,51.67 | v58.52,51.67 54.54,51.67
  Bottom 0.508: v64.48,67.5 64.48,66.05 64.78,65.75
TXD  (via drill 0.1 pad 0.4)
  Top 0.305: U$16.1 65.2,69.29 65.2,70.33 64.98,70.55 v64.34,70.55
  Top 0.4: U$2.TXD 48.82,38.83 49.3,39.3 v50.09,39.3
  Bottom 0.305: 50.82,69.17 51.17,69.52 62.91,69.52 63.93,70.55 v64.34,70.55
  Bottom 0.4: v50.09,39.3 50.07,39.32 50.07,68.42 50.82,69.17 50.91,69.25
VCC  (via drill 0.1 pad 0.4, 0.1 pad 0.8, 0.1 pad 1, 0.2 pad 1)  (2 unrouted)
  Top 0.305: U$3.VDDIO 55.87,51.67 55.49,52.06 55.49,52.8 55.66,52.97 U$3.VDD | IC1.13 53.97,50.71 53.97,50.35 | IC1.8 51.25,49.45 v50.72,48.93 | U$4.2 60.89,52.66 60.63,52.41 60.63,50.39 60.58,50.34
  Top 0.4: U$3.VDDIO 55.54,51.67 | 54.78,50.91 54.61,50.75 54.54,50.75 | 54.78,50.91 55.09,51.22 | 55.09,51.22 55.54,51.67 | 55.54,51.67 55.49,51.72 55.49,52.06 | IC1.13 54.3,50.75 | 54.3,50.75 54.54,50.75 | 54.54,50.75 54.78,50.5 | 55.09,50.2 55.32,49.96 | 57.32,49.96 60,49.96 | 57.32,49.96 56.83,49.96 | 56.83,49.96 56.33,49.96 | 56.33,49.96 55.32,49.96 | 55.09,51.22 55.09,50.2 | 55.09,50.2 54.78,50.5 | 54.78,50.5 54.78,50.91 | 54.3,50.75 54.3,50.44 | 54.3,50.44 54.3,49.92 54.34,49.96 | 54.78,50.5 54.78,50.39 54.34,49.96 | 55.09,50.2 54.55,50.2 54.3,50.44 | 55.32,49.96 54.67,49.96 54.34,49.96 | 56.83,49.96 56.83,49.74 56.83,49.46 | 56.83,49.46 56.33,49.96 | 56.83,49.46 57.32,49.95 57.32,49.96
  Top 0.406: 60,49.96 60.2,49.96 60.58,50.34
  Top 0.5: v56.81,49.74 56.82,49.74 56.83,49.74
  Top 0.508: 47.55,42.84 U$2.VCC | U1.3.3V 37.67,73.06 35.89,74.85 U$30.2 | 42.39,54.04 47.87,54.04 48.6,53.3 48.6,48.13 U$6.1 | 42.39,54.04 41.66,54.04 | 41.66,54.54 41.89,54.54 42.39,54.04 | 41.66,52 41.66,53.31 42.39,54.04 | v53.84,48.94 v53.84,48.93 | 51.36,38 U$2.V3 | U$6.1 | v50.72,48.93 49.93,48.93 U$6.1 | v53.84,48.94 54.09,48.68 | 54.09,48.68 U$9.1 | 54.09,49.38 54.09,50.58 53.97,50.71 | U$9.1 54.12,47.85 U$12.1 U$11.1 | U$9.1 53.84,48.1 v53.84,48.94 | IC1.13 53.97,49.06 v53.84,48.94 | 54.09,48.68 54.09,49.38 | 54.09,49.38 54.67,49.96
  Top 0.61: 51.36,40 51.36,39.14 | 51.36,38 51.36,39 | 51.36,39 50.97,39.39 50.97,40.25 | 51.36,39 51.36,39.14 | 51.36,39.14 52.47,40.25
  Top 1: 41.65,38.97 U$18.2 IC3.VOUT 41.66,44.25 | U$14.2 62.31,41.25 IC2.VOUT 62.33,41.84 | 62.33,45.79 62.33,45.25 61.45,46.13 61.2,46.13 | 62.33,46.92 IC2.VOUT1 60.48,47.07 v60.03,47.52 | 62.33,45 61.2,46.13 | IC3.VOUT1 41.66,44.25 | 41.66,44.25 40.54,45.38 40.54,47.13 41.6,47.13 IC3.VOUT1 | 42.23,44.82 42.78,45.37 42.78,46.73 | 41.66,44.25 42.23,44.82 | 42.23,44.82 42.23,45.7 41.07,45.7 | 62.33,44.25 61.2,45.38 61.2,46.13 | U1.3.3V 44.15,73.06 44.77,72.45 44.77,57.1 43.97,56.3 42.37,56.3 41.66,55.59 41.66,54.54 41.66,54.04 41.66,52 IC3.VOUT1
  Top 1.016: 62.33,41.84 62.33,44.25 | 62.33,45.79 62.33,46.92 | 63.25,45.18 63.45,45.38 63.45,46.59 63.12,46.59 62.33,45.79 | 63.25,45.18 62.33,44.25 | 62.33,44.25 62.33,45.79 | IC2.VOUT1 63.25,46.14 63.25,45.18 | v39.79,51.88 39.79,50.73 37.24,48.19 J3.6 | 61.2,45.38 61.2,44.33 60.12,43.25 59.19,43.25 58.53,42.59 58.53,41.71 57.07,40.25 52.47,40.25 50.97,40.25 47.24,40.25 | 42.23,44.82 43.58,43.47 44.69,43.47 45.27,42.89 | 47.24,40.25 45.75,41.74 45.75,42.41 | 45.75,42.41 45.27,42.89 | U$2.VCC 47.55,41 | 47.55,41 47.55,40.56 47.24,40.25 | U$2.VCC 47.32,42.41 47,42.41 | 47,42.41 45.75,42.41 | 47.55,41 46.68,41.87 46.61,41.87 46.61,42.02 47,42.41 | U$2.VCC 47.3,42.89 45.27,42.89
  Top 1.5: 61.45,46.06 61.45,46.13
  Bottom 0.508: v50.72,48.93 v50.73,48.94 v53.84,48.94
  Bottom 1: v56.81,49.74 58.68,49.74 60.03,48.4 v60.03,47.52 | 60.1,47.52 v60.03,47.52
  Bottom 1.016: v41.65,50.38 41.29,50.38 39.78,51.89
(copper drawn outside any net)
  shapes: Top area x1

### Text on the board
tPlace: GND | IO25 | IO26 | SCL | IO14 | SDA | IO12 | IO19 | B+ | IO18 | VCC | IO5 | IO17 | GND | IO16
bPlace: + | - | - | + | BATTERY | 3.7V | - | - | + | - | + | - | +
